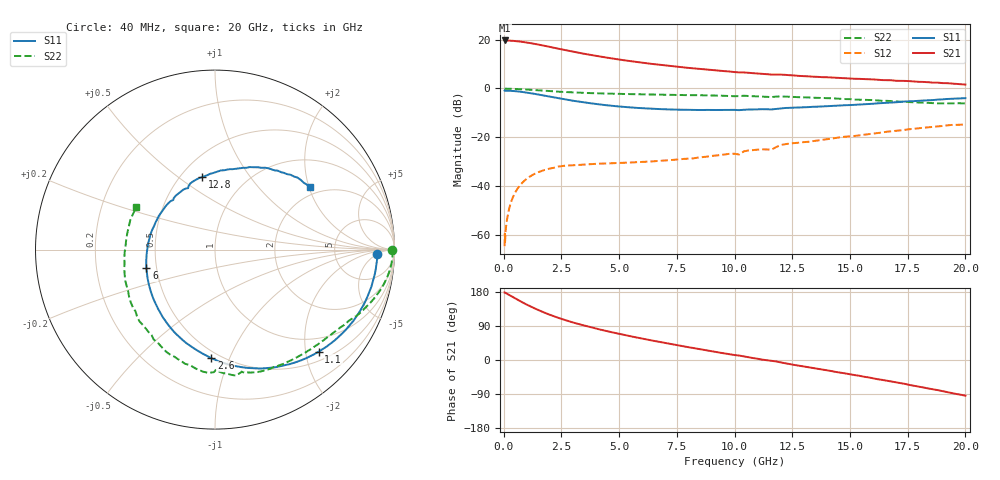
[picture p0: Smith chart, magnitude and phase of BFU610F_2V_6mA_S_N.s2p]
! Filename:  P:\Prog\Test\Noise\ATS_data\Testdata_Net\SplitFiles\BFU610_2W_A5_HighFreq_2V_6mA_D.s2p
! Date/Time: Wed 10/Aug/2011 16:56:05
! BFU610_2W_A5_HighFreq_2V_1mA_10mA_Bias5_R.s2p
! MDIF S-parameter v. bias file
! BFU610_2W_A5_HighFreq_2V_1mA_10mA
! Date/time Mon Aug 08 14:20:39 2011
! VAR V_out= 2.0002
! VAR I_out= 5.9950
! VAR V_in= 0.9085
! VAR I_in= 0.0501
! Device data file deembeded for feedlines and parallel
! Original file: \SplitFiles\BFU610_2W_A5_HighFreq_2V_6mA_R.s2p
! Feed-files: PR003V01_101208_Feed1.s2p, PR003V01_101208_Feed2.s2p
! Parallel-file: PR003V01_101208_Par.s2p
# MHz S MA R 50
!  Freq-MHz  S11-mag  S11-arg  S21-mag  S21-arg  S12-mag  S12-arg  S22-mag  S22-arg
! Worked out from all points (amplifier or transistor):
!   167 points, 40 MHz to 20 GHz, reference 50 ohm
!   highest |S21| = 19.6 dB at 40 MHz (marker M1)
!   |S21| within 3 dB of that: start of sweep to 2.188 GHz
!   unconditionally stable (mu >= 1): 3.885 GHz to 19.17 GHz
!   at 550 MHz: K = 0.10, MSG = 30.5 dB, |S12| = -41.6 dB
!   at 4.2 GHz: K = 1.09, MAG = 20.0 dB, |S12| = -30.7 dB
!   at 20 GHz: K = 0.98, MSG = 8.1 dB, |S12| = -14.7 dB
!   lowest NFmin = 1.35 dB at 400 MHz
!   S11 on the Smith chart (normalised r, x): 40 MHz: 18, -5; 1.1 GHz: 0.68, -2.27; 2.6 GHz: 0.45, -0.86; 6 GHz: 0.44, -0.11; 12.8 GHz: 0.63, +0.62; 20 GHz: 1.76, +2.04
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40  0.9045 -1.6  9.562 178.4  0.0006046 85.4  0.9873 -0.2
50  0.8971 -2.4  9.527 178.4  0.001088 61.8  0.9884 -0.4
60  0.9039 -2.2  9.554 177.5  0.0007344 79.7  0.989 -0.6
140  0.9027 -5.9  9.518 175.0  0.002063 88.8  0.9893 -1.8
320  0.895 -13.6  9.426 168.7  0.00484 84.8  0.9866 -4.3
550  0.877 -23.1  9.277 160.7  0.008291 78.8  0.978 -7.4
750  0.8557 -31.2  9.03 154.0  0.01116 73.6  0.9676 -10.0
1100  0.8107 -44.5  8.519 143.2  0.01555 65.6  0.9459 -14.1
1350  0.7755 -53.5  8.13 135.9  0.01819 60.5  0.9289 -16.8
1750  0.7177 -67.0  7.471 125.4  0.02157 53.5  0.9018 -20.6
2250  0.6503 -82.2  6.67 113.6  0.02451 47.3  0.8709 -25.1
2600  0.6053 -91.9  6.159 106.6  0.02638 42.7  0.8486 -27.6
3400  0.5275 -111.7  5.199 92.4  0.02786 37.0  0.8166 -33.0
4500  0.4524 -135.8  4.241 75.8  0.02959 34.0  0.7876 -40.1
6000  0.3963 -164.8  3.362 56.4  0.03168 34.9  0.7601 -49.9
6800  0.379 -178.8  3.028 47.1  0.03337 36.5  0.7489 -55.3
8600  0.3637 152.6  2.488 27.4  0.03961 41.4  0.7273 -67.7
10200  0.3613 130.0  2.127 11.7  0.04505 45.3  0.699 -78.0
12800  0.4101 100.2  1.807 -15.0  0.07847 38.5  0.6627 -101.2
13400  0.4231 93.8  1.742 -21.0  0.0842 35.8  0.6481 -107.0
16800  0.5188 62.0  1.471 -57.0  0.1337 15.2  0.5531 -148.2
20000  0.6348 33.1  1.203 -94.2  0.1847 -16.8  0.498 151.9
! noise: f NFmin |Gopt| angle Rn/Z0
400  1.348  0.5119  2.714  0.4672
800  1.386  0.4928  6.92  0.4708
1250  1.433  0.4724  11.57  0.4717
1700  1.483  0.4529  16.11  0.4696
2150  1.537  0.4339  20.56  0.4649
2700  1.608  0.4108  25.86  0.4562
3600  1.735  0.3724  34.23  0.437
4500  1.877  0.3316  42.36  0.4144
5800  2.108  0.2659  54.1  0.3827
8000  2.568  0.1316  80.01  0.3573
